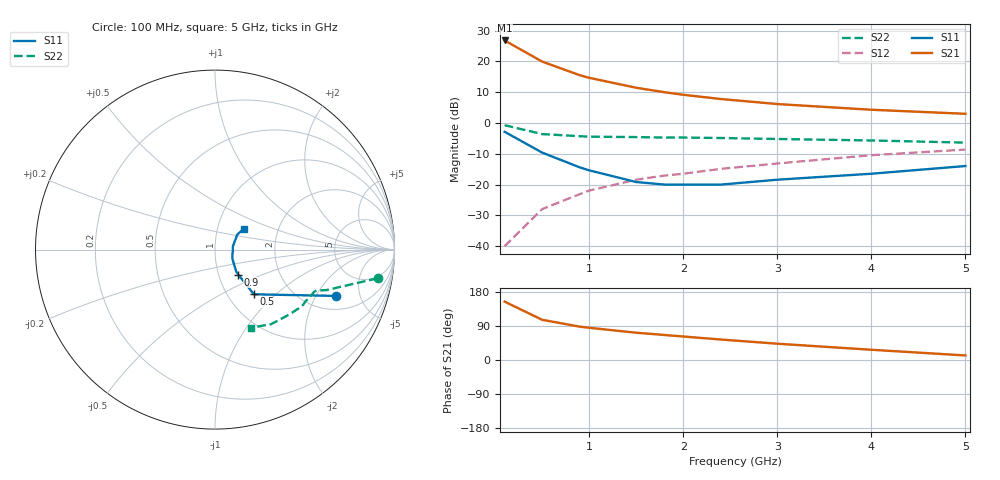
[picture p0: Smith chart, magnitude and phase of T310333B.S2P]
!AT-31033
!S and NOISE PARAMETERS at Vce=2.7V  Ic=10mA.  LAST UPDATED 04-10-94
# ghz s ma r 50
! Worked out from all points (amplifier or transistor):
!   11 points, 100 MHz to 5 GHz, reference 50 ohm
!   highest |S21| = 26.8 dB at 100 MHz (marker M1)
!   |S21| within 3 dB of that: start of sweep to 274.8 MHz
!   unconditionally stable (mu >= 1): 855.2 MHz to 3.473 GHz
!   at 500 MHz: K = 0.91, MSG = 23.9 dB, |S12| = -28.0 dB
!   at 1.8 GHz: K = 1.02, MAG = 12.6 dB, |S12| = -17.1 dB
!   at 5 GHz: K = 0.95, MSG = 5.8 dB, |S12| = -8.6 dB
!   lowest NFmin = 1.30 dB at 500 MHz
!   S11 on the Smith chart (normalised r, x): 100 MHz: 2.77, -2.97; 500 MHz: 1.32, -0.74; 900 MHz: 1.24, -0.36; 5 GHz: 1.34, +0.33
0.1  0.72 -21.0  21.87 154.0  0.01 80.0  0.92 -10.0
0.5  0.33 -49.0  9.92 106.0  0.04 73.0  0.66 -20.0
0.9  0.19 -47.0  5.96 88.0  0.07 72.0  0.61 -22.0
1  0.17 -46.0  5.41 85.0  0.08 72.0  0.6 -23.0
1.5  0.11 -28.0  3.73 72.0  0.12 69.0  0.59 -27.0
1.8  0.1 -14.0  3.16 66.0  0.14 67.0  0.58 -30.0
2  0.1 -6.0  2.87 62.0  0.15 65.0  0.58 -32.0
2.4  0.1 9.0  2.45 54.0  0.18 62.0  0.57 -35.0
3  0.12 23.0  2.03 43.0  0.22 57.0  0.55 -41.0
4  0.15 34.0  1.64 27.0  0.3 48.0  0.52 -53.0
5  0.2 36.0  1.41 12.0  0.37 38.0  0.48 -65.0
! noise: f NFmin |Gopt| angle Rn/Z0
0.5  1.3  0.42  10  0.38
0.9  1.4  0.31  30  0.34
1.8  1.7  0.16  80  0.23
2.4  2  0.08  118  0.17
